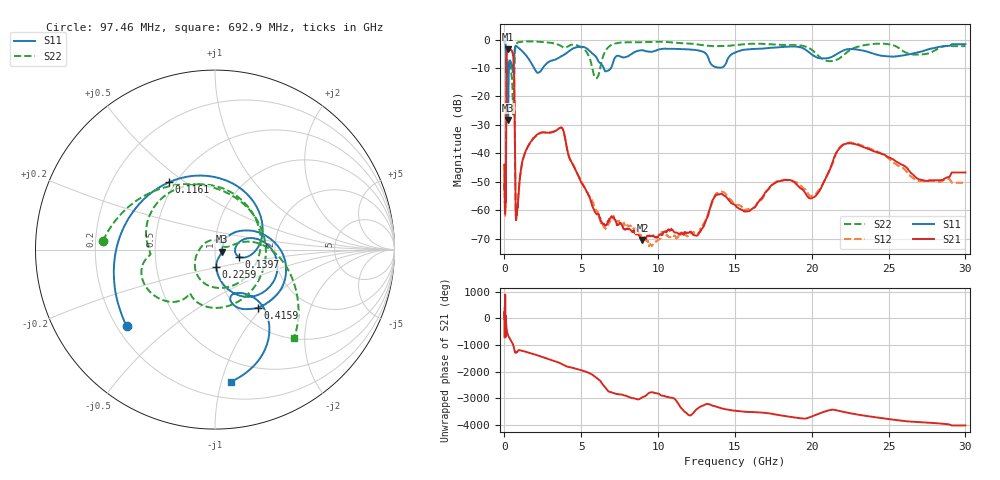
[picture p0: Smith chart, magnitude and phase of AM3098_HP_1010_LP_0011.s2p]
! Date/Time: Thu, Feb 28, 2019 8:41 AM
! Network Analyzer: Agilent Technologies E8364B Rev: A.07.50.67
! Sweep from 0.010 to 30.000 GHz, 1601 Points, Sweep Type: LOG
! Power Supply: 5.023 V, 0.002 A
# Hz S DB R 50
!freq MagS11 AngS11 MagS21 AngS21 MagS12 AngS12 MagS22 AngS22
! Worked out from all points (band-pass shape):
!   1601 points, 10 MHz to 30 GHz, reference 50 ohm
!   highest |S21| = -3.39 dB at 239.9 MHz (marker M1); lowest = -70.3 dB at 8.982 GHz (marker M2)
!   |S21| within 3 dB of the highest: 133.1 MHz to 580.9 MHz (447.9 MHz wide, 125 % of centre)
!   lowest |S11| = -28.3 dB at 238.7 MHz (marker M3), VSWR 1.08, Z = 53.8 - j1.26 ohm
!   |S11| at or under -10 dB: 199.5 MHz to 291.3 MHz (91.81 MHz wide, 37.4 % of centre); 1.921 GHz to 2.497 GHz (575.3 MHz wide, 26 % of centre); 6.462 GHz to 6.935 GHz (472.4 MHz wide, 7.05 % of centre)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
!   |S22| runs from -26.4 to -0.5 dB; largest |S21 - S12| = 0.013
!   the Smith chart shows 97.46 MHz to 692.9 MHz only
!   S11 on the Smith chart (normalised r, x): 97.46 MHz: 0.24, -0.36; 116.1 MHz: 0.46, +0.44; 139.7 MHz: 1.30, -0.11; 225.9 MHz: 1.00, -0.19; 415.9 MHz: 1.22, -0.95; 692.9 MHz: 0.33, -1.07
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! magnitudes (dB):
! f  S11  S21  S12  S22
! 10 MHz  -0.3  -43.9  -43.9  -0.5
! 38.04 MHz  -0.4  -58.7  -59.9  -0.8
! 97.46 MHz  -3.7  -49.2  -49.1  -4.1
! 116.1 MHz  -6.9  -18.7  -18.7  -10.7
! 139.7 MHz  -17.1  -5.2  -5.2  -11.0
! 144.7 MHz  -19.0  -4.8  -4.8  -10.9
! 185.8 MHz  -8.7  -4.0  -4.0  -7.2
! 225.9 MHz  -20.3  -3.5  -3.4  -8.7
! 238.7 MHz  -28.3  -3.4  -3.4  -8.9
! 239.9 MHz  -28.2  -3.4  -3.4  -8.9
! 415.9 MHz  -7.9  -3.7  -3.6  -11.1
! 550.5 MHz  -11.5  -5.1  -5.1  -24.3
! 630.1 MHz  -6.1  -12.9  -12.9  -13.6
! 692.9 MHz  -2.6  -44.8  -44.4  -3.6
! 769.7 MHz  -2.3  -63.0  -61.4  -1.6
! 2.084 GHz  -11.4  -33.6  -33.6  -0.7
! 3.723 GHz  -5.8  -30.9  -31.0  -2.4
! 7.926 GHz  -6.1  -66.7  -65.0  -1.0
! 8.982 GHz  -3.8  -70.3  -69.7  -1.0
! 20 GHz  -5.3  -55.7  -55.0  -3.6
! 22.56 GHz  -3.3  -36.5  -36.2  -3.5
! 30 GHz  -1.7  -46.7  -50.3  -2.3
